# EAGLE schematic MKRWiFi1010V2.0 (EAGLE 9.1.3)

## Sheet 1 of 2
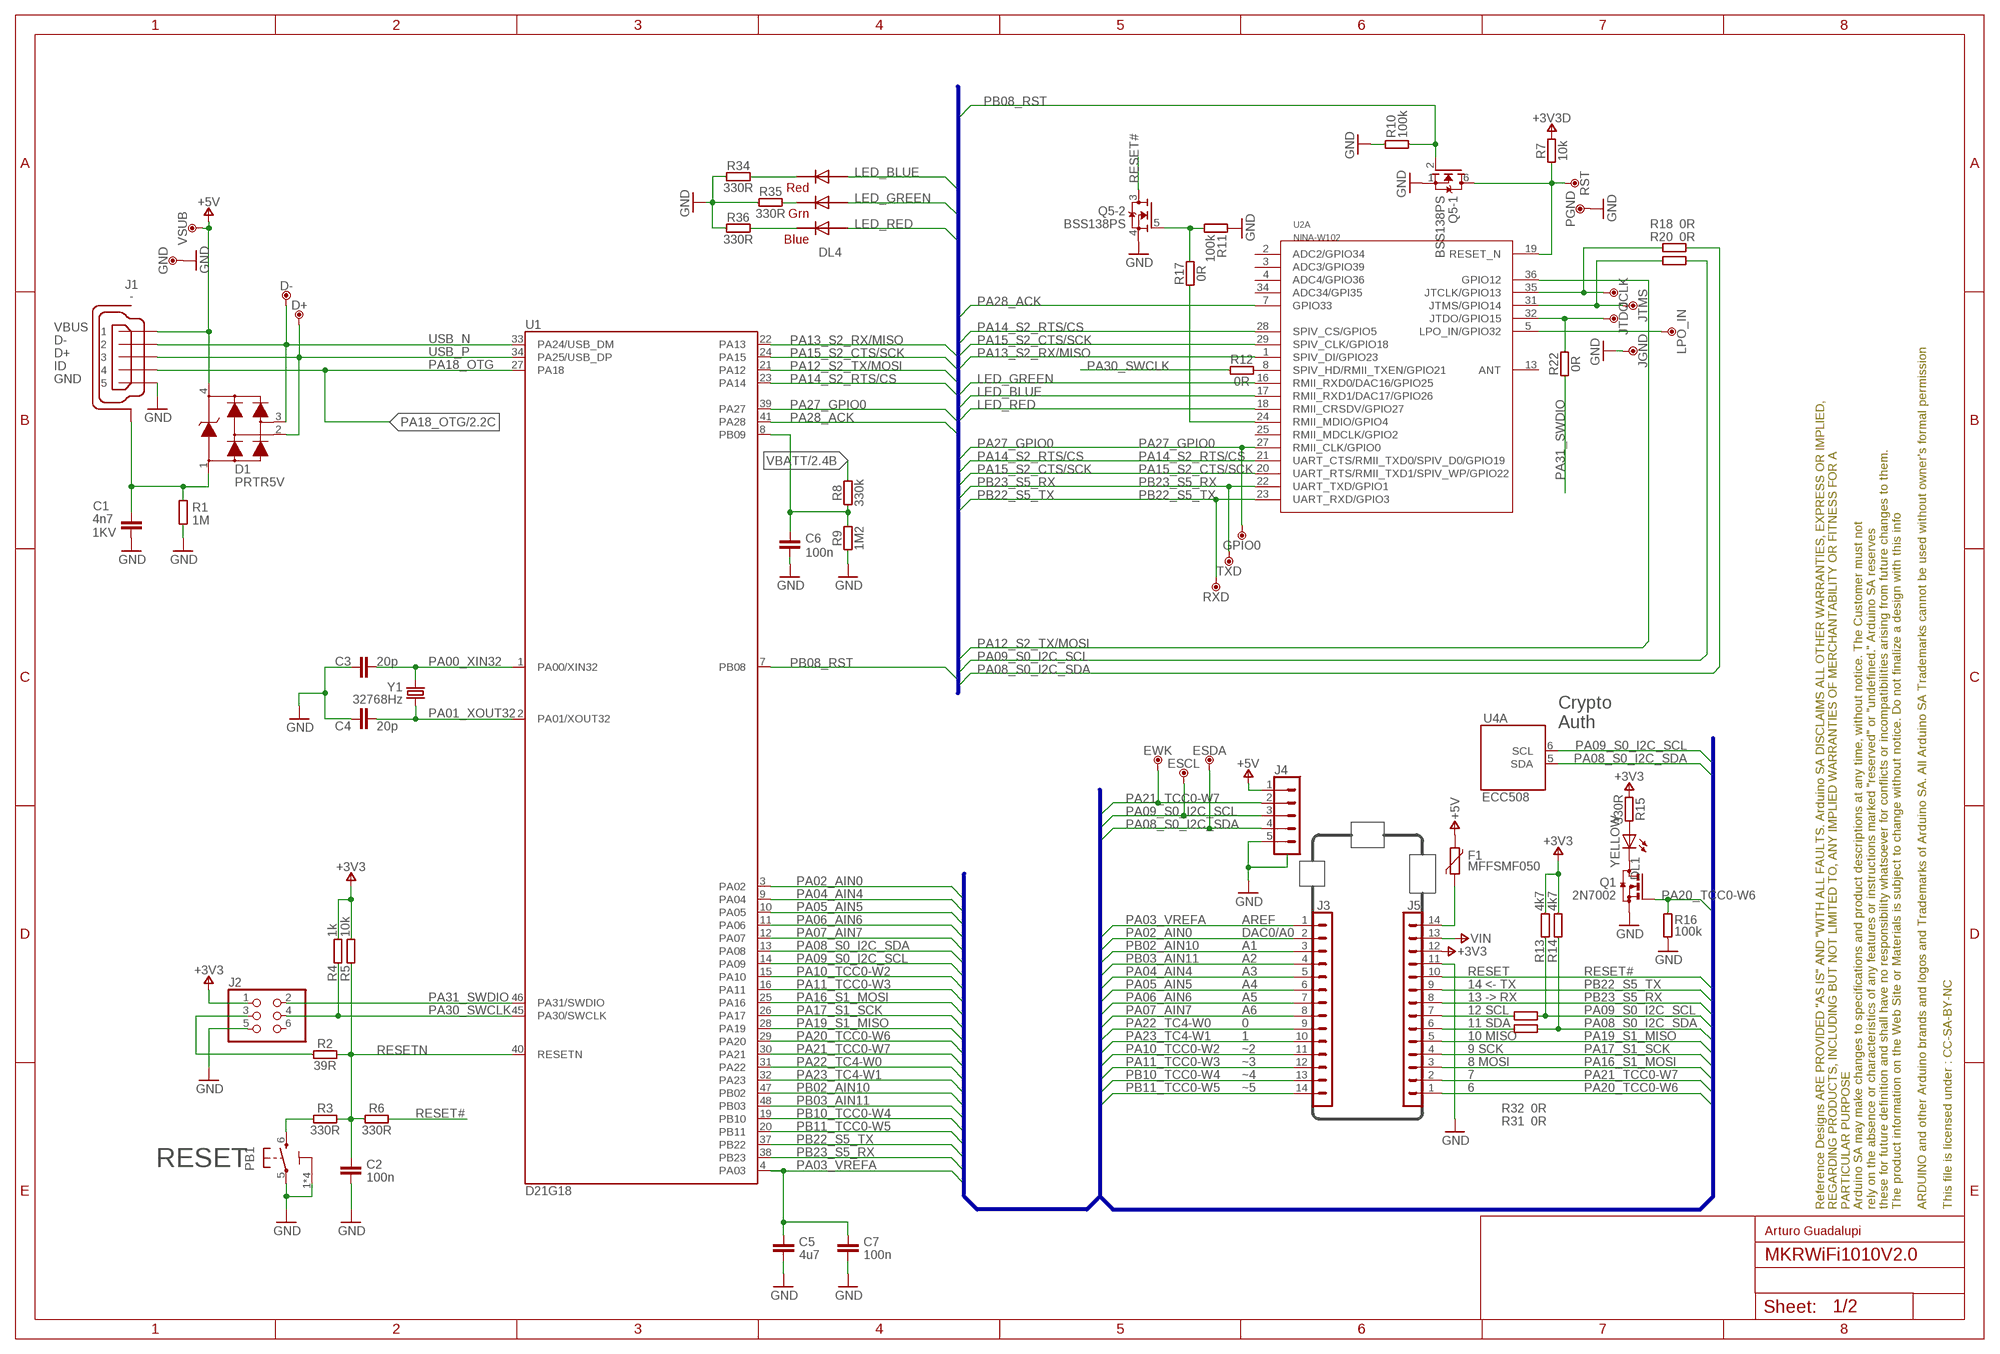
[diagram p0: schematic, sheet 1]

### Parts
C1  4n7  C4.7NF-0805  [0805-R2013X50N]
C2  100n  C-100NF-0402  [0402-1005X55N]
C3  20p  C-20PF-0402  [0402-1005X55N]
C4  20p  C-20PF-0402  [0402-1005X55N]
C5  4u7  C-4.7UF-0402  [0402-1005X55N]
C6  100n  C-100NF-0402  [0402-1005X55N]
C7  100n  C-100NF-0402  [0402-1005X55N]
D1  PRTR5V  PRTR5V0U2X,215  [SOT190P230X110-4N]
D+  DNP  TPTP-1.00MM  [TP-1.00MM]
D-  DNP  TPTP-1.00MM  [TP-1.00MM]
DL1  YELLOW  LED-YELLOW-0603  [LEDC1608X80N-AK]
DL4  RGB  RGBLED5050  [RGBLED]
ESCL  DNP  TPTP-1.00MM  [TP-1.00MM]
ESDA  DNP  TPTP-1.00MM  [TP-1.00MM]
EWK  DNP  TPTP-1.00MM  [TP-1.00MM]
F1  MFFSMF050  PTC  [0603-1608X90N]
FRAME1  DNP  A3-FRAME-STANDARD  [FRAME]
GND  DNP  TPTP-1.00MM  [TP-1.00MM]
GPIO0  DNP  TPTP-0.8MM  [TP-0.8MM]
J1  -  USB-MICRO  [ZX62-AB-5PA]
J2  DNP  PINHD-2X03-DNPSMD-NH  [2X3_SMT]
J3  -  PINHD-1X14-SM-MALE/FEMALETH-SMD  [1X14_SMD_TH]
J4  -  SM05B-SRSS-TB  [SM05B-SRSS-TB]
J5  -  PINHD-1X14-SM-MALE/FEMALETH-SMD  [1X14_SMD_TH]
JCLK  DNP  TPTP-0.8MM  [TP-0.8MM]
JGND  DNP  TPTP-0.8MM  [TP-0.8MM]
JTDO  DNP  TPTP-0.8MM  [TP-0.8MM]
JTMS  DNP  TPTP-0.8MM  [TP-0.8MM]
LPO_IN  DNP  TPTP-1.27MM  [TP-1.27MM]
PB1  PTS820  TACTILE1PTS820-NH  [C&K_PTS820_NO_HOLES]
PGND  DNP  TPTP-0.8MM  [TP-0.8MM]
Q1  2N7002  2N7002T-SOT523  [SOTFL50P160X78-3]
Q5  BSS138PS  [SOT363]
R1  1M  R-1M-0402  [0402-1005X55N]
R2  39R  R-39R-0402  [0402-1005X55N]
R3  330R  R-330R-0402  [0402-1005X55N]
R4  1k  R-1K-0402  [0402-1005X55N]
R5  10k  R-10K-0402  [0402-1005X55N]
R6  330R  R-330R-0402  [0402-1005X55N]
R7  10k  R-10K-0402  [0402-1005X55N]
R8  330k  R-330K-0402  [0402-1005X55N]
R9  1M2  R-1M2-0402  [0402-1005X55N]
R10  100k  R-100K-0402  [0402-1005X55N]
R11  100k  R-100K-0402  [0402-1005X55N]
R12  0R  R-0R-0402  [0402-1005X55N]
R13  4k7  R-4K7-0402  [0402-1005X55N]
R14  4k7  R-4K7-0402  [0402-1005X55N]
R15  330R  R-330R-0402  [0402-1005X55N]
R16  100k  R-100K-0402  [0402-1005X55N]
R17  0R  R-0R-0402  [0402-1005X55N]
R18  0R  R-0R-0402  [0402-1005X55N]
R20  0R  R-0R-0402  [0402-1005X55N]
R22  0R  R-0R-0402  [0402-1005X55N]
R31  0R  R-0R-0402  [0402-1005X55N]
R32  0R  R-0R-0402  [0402-1005X55N]
R34  330R  R-330R-0402  [0402-1005X55N]
R35  330R  R-330R-0402  [0402-1005X55N]
R36  330R  R-330R-0402  [0402-1005X55N]
RST  DNP  TPTP-0.8MM  [TP-0.8MM]
RXD  DNP  TPTP-0.8MM  [TP-0.8MM]
TXD  DNP  TPTP-0.8MM  [TP-0.8MM]
U1  D21G18  ATSAMD21G18A-48QFN  [QFN50P700X700X90-49XN-EPSQ515]
U2  NINA-W102  NINA-W1X-102  [NINA-W1X]
U4  ECC508  ATECC508A-MAHDA-T8-UDFN  [SON50P300X200X60-9N-EP160X140]
VSUB  DNP  TPTP-1.00MM  [TP-1.00MM]
Y1  32768Hz  32.768KHZ  [ABS07]

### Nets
+3V3: J2.1 J5.12 R4.2 R5.2 R13.2 R14.2 R15.1 ; also sheet 2
+3V3D: R7.2 ; also sheet 2
+5V: D1.4 F1.2 J1.1 J4.1 VSUB.X ; also sheet 2
GND: C1.2 C2.2 C3.1 C4.1 C5.2 C6.2 C7.2 GND.X J1.5 J2.5 J4.5 J4.SH1(SH) J4.SH2(SH) J5.11 JGND.X PB1.1 PB1.2 PB1.3 PB1.4 PB1.5 PGND.X Q1.S Q5.1(-1:S) Q5.4(-2:S) R1.1 R9.1 R10.2 R11.2 R16.1 R34.1 R35.1 R36.1 ; also sheet 2
LED_BLUE: DL4.2(RED_A) U2.17(A:RMII_RXD1/DAC17/GPIO26)
LED_GREEN: DL4.1(GREEN_A) U2.16(A:RMII_RXD0/DAC16/GPIO25)
LED_RED: DL4.3(BLUE_A) U2.18(A:RMII_CRSDV/GPIO27)
N17658775: PB1.6 R3.1
N$1: C1.1 D1.1 J1.6(SH) J1.7(SH) J1.8(SH) J1.9(SH) J1.10(SH) J1.11(SH) R1.2
N$2: F1.1 J5.14
N$4: J2.3 R2.1
N$5: J5.7 R32.1
N$6: C6.1 R8.1 R9.2 U1.8(PB09)
N$7: DL1.A R15.2
N$8: J5.6 R31.1
N$9: Q5.6(-1:D) R7.1 RST.X U2.19(A:RESET_N)
N$10: DL1.C Q1.D
N$11: JCLK.X R18.1 U2.35(A:JTCLK/GPIO13)
N$12: JTMS.X R20.1 U2.31(A:JTMS/GPIO14)
N$13: R17.1 U2.24(A:RMII_MDIO/GPIO4)
N$14: DL4.5(RED_C) R34.2
N$16: DL4.6(GREEN_C) R35.2
N$20: DL4.4(BLUE_C) R36.2
N$25: LPO_IN.X U2.5(A:LPO_IN/GPIO32)
N$26: JTDO.X R22.2 U2.32(A:JTDO/GPIO15)
N$27: R12.2 U2.8(A:SPIV_HD/RMII_TXEN/GPIO21)
N$28: Q5.5(-2:G) R11.1 R17.2
PA00_XIN32: C3.2 U1.1(PA00/XIN32) Y1.2
PA01_XOUT32: C4.2 U1.2(PA01/XOUT32) Y1.1
PA02_AIN0: J3.2 U1.3(PA02)
PA03_VREFA: C5.1 C7.1 J3.1 U1.4(PA03)
PA04_AIN4: J3.5 U1.9(PA04)
PA05_AIN5: J3.6 U1.10(PA05)
PA06_AIN6: J3.7 U1.11(PA06)
PA07_AIN7: J3.8 U1.12(PA07)
PA08_S0_I2C_SDA: ESDA.X J4.4 R14.1 R18.2 R31.2 U1.13(PA08) U4.5(A:SDA) ; also sheet 2
PA09_S0_I2C_SCL: ESCL.X J4.3 R13.1 R20.2 R32.2 U1.14(PA09) U4.6(A:SCL) ; also sheet 2
PA10_TCC0-W2: J3.11 U1.15(PA10)
PA11_TCC0-W3: J3.12 U1.16(PA11)
PA12_S2_TX/MOSI: U1.21(PA12) U2.36(A:GPIO12)
PA13_S2_RX/MISO: U1.22(PA13) U2.1(A:SPIV_DI/GPIO23)
PA14_S2_RTS/CS: U1.23(PA14) U2.21(A:UART_CTS/RMII_TXD0/SPIV_D0/GPIO19) U2.28(A:SPIV_CS/GPIO5)
PA15_S2_CTS/SCK: U1.24(PA15) U2.20(A:UART_RTS/RMII_TXD1/SPIV_WP/GPIO22) U2.29(A:SPIV_CLK/GPIO18)
PA16_S1_MOSI: J5.3 U1.25(PA16)
PA17_S1_SCK: J5.4 U1.26(PA17)
PA18_OTG: J1.4 U1.27(PA18) ; also sheet 2
PA19_S1_MISO: J5.5 U1.28(PA19)
PA20_TCC0-W6: J5.1 Q1.G R16.2 U1.29(PA20)
PA21_TCC0-W7: EWK.X J4.2 J5.2 U1.30(PA21)
PA22_TC4-W0: J3.9 U1.31(PA22)
PA23_TC4-W1: J3.10 U1.32(PA23)
PA27_GPIO0: GPIO0.X U1.39(PA27) U2.27(A:RMII_CLK/GPIO0)
PA28_ACK: U1.41(PA28) U2.7(A:GPIO33)
PA30_SWCLK: J2.4 R4.1 R12.1 U1.45(PA30/SWCLK)
PA31_SWDIO: J2.2 R22.1 U1.46(PA31/SWDIO)
PB02_AIN10: J3.3 U1.47(PB02)
PB03_AIN11: J3.4 U1.48(PB03)
PB08_RST: Q5.2(-1:G) R10.1 U1.7(PB08)
PB10_TCC0-W4: J3.13 U1.19(PB10)
PB11_TCC0-W5: J3.14 U1.20(PB11)
PB22_S5_TX: J5.9 RXD.X U1.37(PB22) U2.23(A:UART_RXD/GPIO3)
PB23_S5_RX: J5.8 TXD.X U1.38(PB23) U2.22(A:UART_TXD/GPIO1)
RESET#: J5.10 Q5.3(-2:D) R6.2
RESETN: C2.1 R2.2 R3.2 R5.1 R6.1 U1.40(RESETN)
USB_N [usb]: D1.3 D-.X J1.2 U1.33(PA24/USB_DM)
USB_P [usb]: D1.2 D+.X J1.3 U1.34(PA25/USB_DP)
VBATT: R8.2 ; also sheet 2
VIN: J5.13 ; also sheet 2
Unconnected: J2.6 U2.2(A:ADC2/GPIO34) U2.3(A:ADC3/GPIO39) U2.4(A:ADC4/GPIO36) U2.13(A:ANT) U2.25(A:RMII_MDCLK/GPIO2) U2.34(A:ADC34/GPI35)

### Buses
PA03_VREFA,PA02_AIN0,PB02_AIN10,PB03_AIN11,PA04_AIN4,PA05_AIN5,PA06_AIN6,PA07_AIN7,PA22_TC4-W0,PA23_TC4-W1,PA10_TCC0-W2,PA11_TCC0-W3,PB10_TCC0-W4,PB11_TCC0-W5,PA20_TCC0-W6,PA21_TCC0-W7,PA16_S1_MOSI,PA17_S1_SCK,PA19_S1_MISO,PA08_S0_I2C_SDA,PA09_S0_I2C_SCL,PB23_S5_RX,PB22_S5_TX,RESET#
B$2

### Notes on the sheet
- Crypto
  Auth
- AREF
- DAC0/A0
- A1
- A2
- A3 | RESET
- A4 | 14 <- TX
- A5 | 13 -> RX
- A6 | 12 SCL
- 0 | 11 SDA
- 1 | 10 MISO
- ~2 | 9 SCK
- ~3 | 8 MOSI
- ~4 | 7
- ~5 | 6
- RESET
- Arturo Guadalupi

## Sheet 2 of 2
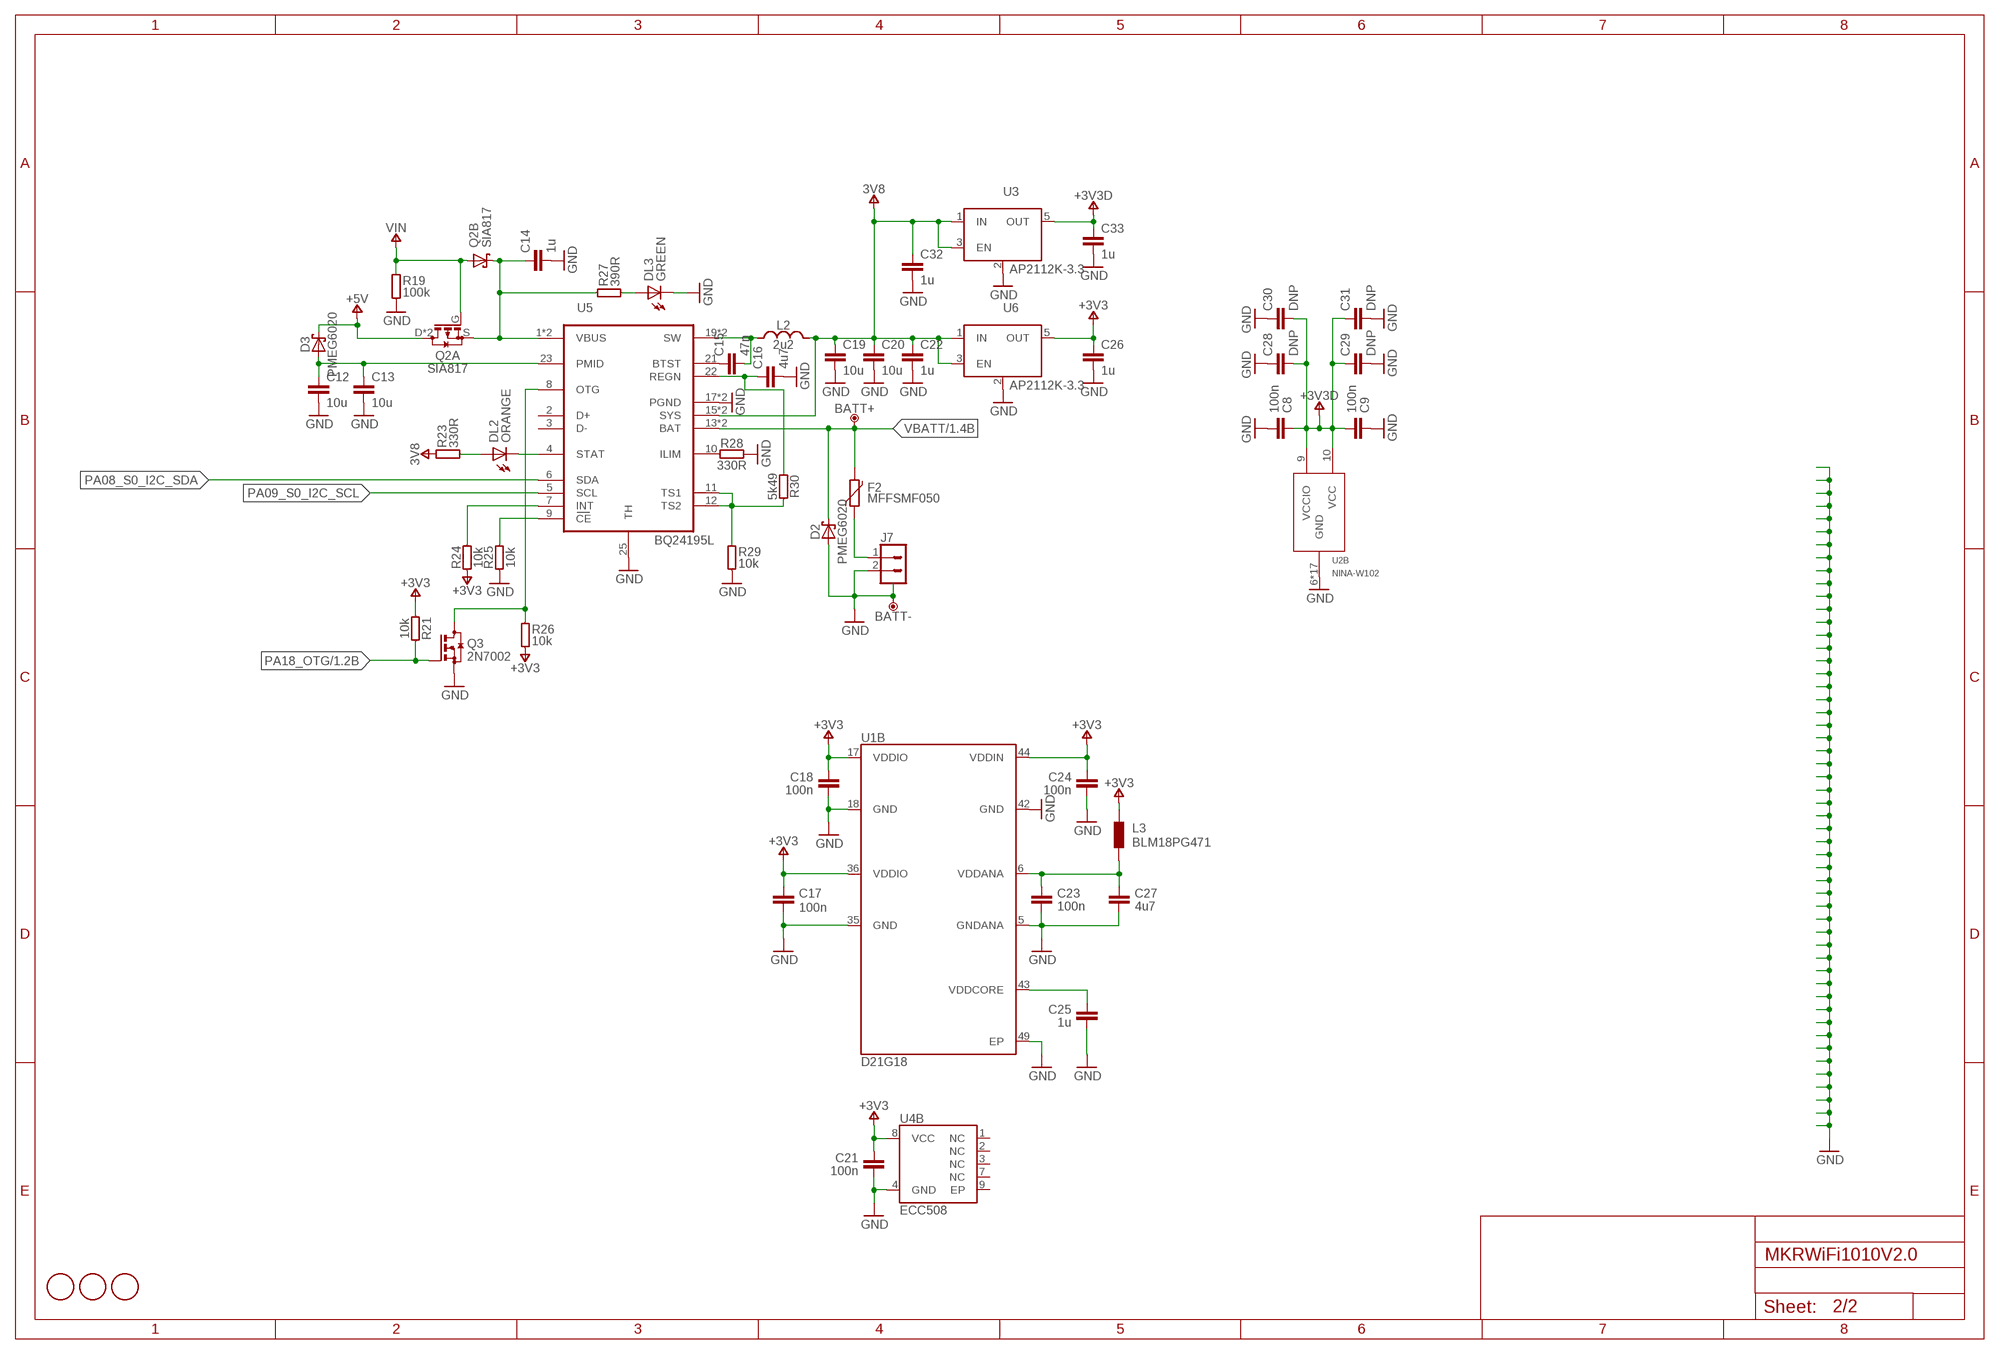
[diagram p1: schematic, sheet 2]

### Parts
BATT+  DNP  TPTP-1.00MM  [TP-1.00MM]
BATT-  DNP  TPTP-1.00MM  [TP-1.00MM]
C8  100n  C-100NF-0402  [0402-1005X55N]
C9  100n  C-100NF-0402  [0402-1005X55N]
C12  10u  C-10UF-0603  [0603-1608X90N]
C13  10u  C-10UF-0603  [0603-1608X90N]
C14  1u  C-1UF-0402  [0402-1005X55N]
C15  47n  C-47N-0402  [0402-1005X55N]
C16  4u7  C-4.7UF-0402  [0402-1005X55N]
C17  100n  C-100NF-0402  [0402-1005X55N]
C18  100n  C-100NF-0402  [0402-1005X55N]
C19  10u  C-10UF-0603  [0603-1608X90N]
C20  10u  C-10UF-0603  [0603-1608X90N]
C21  100n  C-100NF-0402  [0402-1005X55N]
C22  1u  C-1UF-0402  [0402-1005X55N]
C23  100n  C-100NF-0402  [0402-1005X55N]
C24  100n  C-100NF-0402  [0402-1005X55N]
C25  1u  C-1UF-0402  [0402-1005X55N]
C26  1u  C-1UF-0402  [0402-1005X55N]
C27  4u7  C-4.7UF-0603  [0603-1608X90N]
C28  DNP  CDNP-0402  [0402-1005X55N]
C29  DNP  CDNP-0402  [0402-1005X55N]
C30  DNP  C-DNP-0603  [0603-1608X90N]
C31  DNP  C-DNP-0603  [0603-1608X90N]
C32  1u  C-1UF-0402  [0402-1005X55N]
C33  1u  C-1UF-0402  [0402-1005X55N]
D2  PMEG6020  PMEG6020AELRX  [SODFL3517X110N]
D3  PMEG6020  PMEG6020AELRX  [SODFL3517X110N]
DL2  ORANGE  LED-ORANGE-0603  [LEDC1608X80N-AK]
DL3  GREEN  LED-GREEN-0603  [LEDC1608X80N-AK]
F2  MFFSMF050  PTC  [0603-1608X90N]
FD1  DNP  FIDUCIAL-1.5MM  [FD-1-1.5]
FD2  DNP  FIDUCIAL-1.5MM  [FD-1-1.5]
FD3  DNP  FIDUCIAL-1.5MM  [FD-1-1.5]
FRAME2  A3-FRAMEONLY  [FRAME-NO-BAN-FRAMEONLY]
J7  -  BATTERY  [JST-S2B-PH-SM4-TB]
L2  2u2  LSRP  [SRP4020]
L3  BLM18PG471  FERRITE-470R0603  [0603-1608X90N]
Q2  SIA817  SIA817EDJ  [SON65P205X205X75-8N-MWSD]
Q3  2N7002  2N7002T-SOT523  [SOTFL50P160X78-3]
R19  100k  R-100K-0402  [0402-1005X55N]
R21  10k  R-10K-0402  [0402-1005X55N]
R23  330R  R-330R-0402  [0402-1005X55N]
R24  10k  R-10K-0402  [0402-1005X55N]
R25  10k  R-10K-0402  [0402-1005X55N]
R26  10k  R-10K-0402  [0402-1005X55N]
R27  390R  R-390R-0402  [0402-1005X55N]
R28  330R  R-330R-0402  [0402-1005X55N]
R29  10k  R-10K-0402  [0402-1005X55N]
R30  5k49  R-5K49-0402  [0402-1005X55N]
U3  AP2112K-3.3  [SOT25]
U5  BQ24195L  BQ24195QFN-24  [QFN24]
U6  AP2112K-3.3  [SOT25]

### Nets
+3V3: C17.1 C18.1 C21.1 C24.1 C26.1 L3.1 R21.1 R24.1 R26.1 U1.17(VDDIO) U1.36(VDDIO) U1.44(VDDIN) U4.8(B:VCC) U6.5(OUT) ; also sheet 1
+3V3D: C8.1 C9.2 C28.2 C29.1 C30.2 C31.1 C33.1 U2.9(B:VCCIO) U2.10(B:VCC) U3.5(OUT) ; also sheet 1
+3V8: C19.1 C20.1 C22.1 C32.1 L2.2 R23.2 U3.1(IN) U3.3(EN) U5.15(SYS) U5.16(SYS) U6.1(IN) U6.3(EN) ; supply symbol labelled 3V8
+5V: D3.C Q2.D2(A:D) Q2.D(A:D) ; also sheet 1
GND: BATT-.X C8.2 C9.1 C12.2 C13.2 C14.2 C16.2 C17.2 C18.2 C19.2 C20.2 C21.2 C22.2 C23.2 C24.2 C25.2 C26.2 C27.2 C28.1 C29.2 C30.1 C31.2 C32.2 C33.2 D2.A DL3.C J7.2 J7.3(SH) J7.4(SH) Q3.S R19.1 R25.1 R28.2 R29.1 U1.5(GNDANA) U1.18(GND) U1.35(GND) U1.42(GND) U1.49(EP) U2.6(B:GND) U2.12(B:GND) U2.14(B:GND) U2.26(B:GND) U2.30(B:GND) U2.GND@1(B:GND) U2.GND@2(B:GND) U2.GND@3(B:GND) U2.GND@4(B:GND) U2.GND@5(B:GND) U2.GND@6(B:GND) U2.GND@7(B:GND) U2.GND@8(B:GND) U2.GND@9(B:GND) U2.GND@10(B:GND) U2.GND@11(B:GND) U2.GND@12(B:GND) U3.2(GND/ADJ) U4.4(B:GND) U5.17(PGND) U5.18(PGND) U5.25(TH) U6.2(GND/ADJ) ; also sheet 1
N17798864: DL2.A R23.1
N17834267: DL3.A R27.1
N17852357: C23.1 C27.1 L3.2 U1.6(VDDANA)
N17852431: C25.1 U1.43(VDDCORE)
N$3: F2.1 J7.1
N$15: C15.2 L2.1 U5.19(SW) U5.20(SW)
N$17: C14.1 Q2.K2(B:C) Q2.K(B:C) Q2.S(A:S) R27.2 U5.1(VBUS) U5.24(VBUS)
N$18: C15.1 U5.21(BTST)
N$19: R28.1 U5.10(ILIM)
N$21: C16.1 R30.1 U5.22(REGN)
N$22: Q3.D R26.2 U5.8(OTG)
N$23: R29.2 R30.2 U5.11(TS1) U5.12(TS2)
N$24: R25.2 U5.9(CE)
PA08_S0_I2C_SDA: U5.6(SDA) ; also sheet 1
PA09_S0_I2C_SCL: U5.5(SCL) ; also sheet 1
PA18_OTG: Q3.G R21.2 ; also sheet 1
PMICINT: R24.2 U5.7(INT)
STAT: DL2.C U5.4(STAT)
VBATT: BATT+.X D2.C F2.2 U5.13(BAT) U5.14(BAT) ; also sheet 1
VIN: Q2.A(B:A) Q2.G(A:G) R19.2 ; also sheet 1
VUSB1: C12.1 C13.1 D3.A U5.23(PMID)
Unconnected: U4.1(B:NC) U4.2(B:NC) U4.3(B:NC) U4.7(B:NC) U4.9(B:EP) U5.2(D+) U5.3(D-)

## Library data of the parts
BATT+ BATT- D+ D- ESCL ESDA EWK GND GPIO0 JCLK JGND JTDO JTMS LPO_IN PGND RST RXD TXD VSUB = Arduino-utility:TP: Testpoint; CODE-ARDUINO: DNP; DATASHEET: DNP; DISTRIBUTOR-LINK: DNP; DISTRIBUTOR-PN: DNP; MANUFACTURER: DNP; MANUFACTURER-PN: DNP
C1 = Arduino-rcl:C: SMD Capacitor; CODE-ARDUINO: 0689; DATASHEET: http://www.kemet.com/Lists/ProductCatalog/Attachments/40/KEM_C1010_X7R_HV_SMD.pdf; DISTRIBUTOR-LINK: www.kemet.com/docfinder?Partnumber=C0805C472KDRACTU; DISTRIBUTOR-PN: 399-6738-1-ND; MANUFACTURER: Kemet; MANUFACTURER-PN: C0805C472KDRACTU; VOLTAGE: 1KV
C2 C6-C9 C17 C18 C21 C23 C24 = Arduino-rcl:C: SMD Capacitor; CODE-ARDUINO: 0132; DATASHEET: http://www.tdk.com/pdf/TDKMLCCCapRange.pdf; DISTRIBUTOR-LINK: http://www.digikey.com/product-detail/en/tdk-corporation/C1005X5R1H104K050BB/445-5942-1-ND/2443982; DISTRIBUTOR-PN: 445-5942-1-ND; MANUFACTURER: TDK; MANUFACTURER-PN: C1005X5R1H104K050BB
C3 C4 = Arduino-rcl:C: SMD Capacitor; CODE-ARDUINO: 2188; DATASHEET: http://www.kemet.com/docfinder?Partnumber=CBR04C200J5GAC; DISTRIBUTOR-LINK: http://www.digikey.com/product-detail/en/kemet/CBR04C200J5GAC/399-6173-1-ND/2732143; DISTRIBUTOR-PN: 399-6173-1-ND; MANUFACTURER: Kemet; MANUFACTURER-PN: CBR04C200J5GAC
C5 C16 = Arduino-rcl:C: SMD Capacitor; CODE-ARDUINO: 0833; DATASHEET: http://search.murata.co.jp/Ceramy/image/img/A01X/partnumbering_e_01.pdf; DISTRIBUTOR-LINK: http://www.digikey.com/product-detail/en/murata-electronics-north-america/GRM155R60J475ME47D/490-5915-1-ND/3719860; DISTRIBUTOR-PN: 490-5915-1-ND; MANUFACTURER: Murata; MANUFACTURER-PN: GRM155R60J475ME47D
C12 C13 C19 C20 = Arduino-rcl:C: SMD Capacitor; CODE-ARDUINO: 2213; DATASHEET: http://www.murata.com/~/media/webrenewal/support/library/catalog/products/capacitor/mlcc/c02e.pdf; DISTRIBUTOR-LINK: http://www.digikey.com/product-search/en?keywords=490-10728-1-ND; DISTRIBUTOR-PN: 490-10728-1-ND; MANUFACTURER: Murata; MANUFACTURER-PN: GRM188R61C106KAALD
C14 C22 C25 C26 C32 C33 = Arduino-rcl:C: SMD Capacitor; CODE-ARDUINO: -; DATASHEET: http://search.murata.co.jp/Ceramy/image/img/A01X/partnumbering_e_01.pdf; DISTRIBUTOR-LINK: http://www.digikey.com/product-detail/en/murata-electronics-north-america/GRM155R61E105KA12D/490-10017-1-ND/5026367; DISTRIBUTOR-PN: 490-10017-1-ND; MANUFACTURER: Murata; MANUFACTURER-PN: GRM155R61E105KA12D
C15 = Arduino-rcl:C: SMD Capacitor; CODE-ARDUINO: 2216; DATASHEET: http://www.murata.com/~/media/webrenewal/support/library/catalog/products/capacitor/mlcc/c02e.pdf; DISTRIBUTOR-LINK: https://www.digikey.com/product-detail/en/murata-electronics-north-america/GRM155R71E473KA88D/490-3254-1-ND/702795; DISTRIBUTOR-PN: 490-3254-1-ND; MANUFACTURER: Murata; MANUFACTURER-PN: GRM155R71E473KA88D
C27 = Arduino-rcl:C: SMD Capacitor; CODE-ARDUINO: 0458; DATASHEET: http://www.murata.com/~/media/webrenewal/support/library/catalog/products/capacitor/mlcc/c02e.pdf; DISTRIBUTOR-LINK: http://www.digikey.com/product-search/en?keywords=490-7203-1-ND; DISTRIBUTOR-PN: 490-7203-1-ND; MANUFACTURER: Murata; MANUFACTURER-PN: GRM188R61E475KE11D
C28-C31 = Arduino-rcl:C: SMD Capacitor; CODE-ARDUINO: DNP; DATASHEET: DNP; DISTRIBUTOR-LINK: DNP; DISTRIBUTOR-PN: DNP; MANUFACTURER: DNP; MANUFACTURER-PN: DNP
D1 = Arduino-diodes:PRTR5V0U2X,215: USB ESD protection; CODE-ARDUINO: 2209; DATASHEET: http://www.nxp.com/documents/data_sheet/PRTR5V0U2X.pdf; DISTRIBUTOR-LINK: http://www.digikey.com/product-detail/en/nxp-semiconductors/PRTR5V0U2X,215/568-4140-1-ND/1589981; DISTRIBUTOR-PN: 568-4140-1-ND; MANUFACTURER: NXP; MANUFACTURER-PN: PRTR5V0U2X,215
D2 D3 = Arduino-diodes:PMEG6020AELRX: 60 V, 2 A low leakage current Schottky barrier rectifier; CODE-ARDUINO: 2208; DATASHEET: http://www.nxp.com/documents/data_sheet/PMEG6020AELR.pdf; DISTRIBUTOR-LINK: http://www.digikey.com/products/en?keywords=%20568-12710-1-ND; DISTRIBUTOR-PN: 568-12710-1-ND; MANUFACTURER: NXP; MANUFACTURER-PN: PMEG6020AELRX
DL1 = Arduino-diodes:LED: LED; CODE-ARDUINO: 2243; DATASHEET: http://media.digikey.com/pdf/Data%20Sheets/Avago%20PDFs/HSMz-Czzz.pdf; DISTRIBUTOR-LINK: http://www.digikey.com/product-detail/en/broadcom-limited/HSMY-C190/516-1424-1-ND/637748; DISTRIBUTOR-PN: 516-1424-1-ND; MANUFACTURER: Avago; MANUFACTURER-PN: HSMY-C190
DL2 = Arduino-diodes:LED: LED; CODE-ARDUINO: 2207; DATASHEET: http://media.digikey.com/pdf/Data%20Sheets/Avago%20PDFs/HSMz-Czzz.pdf; DISTRIBUTOR-LINK: http://www.digikey.com/product-detail/en/broadcom-limited/HSMD-C190/516-2489-1-ND/2744915; DISTRIBUTOR-PN: 516-2489-1-ND; MANUFACTURER: Avago; MANUFACTURER-PN: HSMD-C190
DL3 = Arduino-diodes:LED: LED; CODE-ARDUINO: 2204; DATASHEET: http://media.digikey.com/pdf/Data%20Sheets/Avago%20PDFs/HSMz-Czzz.pdf; DISTRIBUTOR-LINK: http://www.digikey.com/product-detail/en/broadcom-limited/HSMG-C190/516-1425-1-ND/637749; DISTRIBUTOR-PN: 516-1425-1-ND; MANUFACTURER: Avago; MANUFACTURER-PN: HSMG-C190
DL4 = Arduino-diodes:RGBLED: 5050 RGB LED; CODE-ARDUINO: 2211; DATASHEET: http://www.osram-os.com/Graphics/XPic9/00134830_0.pdf; DISTRIBUTOR-LINK: https://www.digikey.com/product-detail/en/osram-opto-semiconductors-inc/LTRBGFSF-ABCB-QKYO-Z/475-2899-1-ND/2415091; DISTRIBUTOR-PN: 475-2899-1-ND; MANUFACTURER: OSRAM Opto Semiconductors Inc.; MANUFACTURER-PN: LTRBGFSF-ABCB-QKYO-Z
F1 F2 = Arduino-rcl:PTC: SMD PTC; CODE-ARDUINO: 2217; DATASHEET: http://www.bourns.com/docs/Product-Datasheets/mffsmf.pdf; DISTRIBUTOR-LINK: http://www.digikey.com/product-detail/en/bourns-inc/MF-FSMF050X-2/MF-FSMF050X-2CT-ND/2039389; DISTRIBUTOR-PN: MF-FSMF050X-2CT-ND; MANUFACTURER: Bourns Inc; MANUFACTURER-PN: MF-FSMF050X-2
FD1-FD3 = Arduino-utility:FIDUCIAL: Fiducial mount; CODE-ARDUINO: DNP; DATASHEET: DNP; DISTRIBUTOR-LINK: DNP; DISTRIBUTOR-PN: DNP; MANUFACTURER: DNP; MANUFACTURER-PN: DNP
FRAME1 = Arduino-utility:A3-FRAME: Schematic frame; CODE-ARDUINO: DNP; DATASHEET: DNP; DISTRIBUTOR-LINK: DNP; DISTRIBUTOR-PN: DNP; MANUFACTURER: DNP; MANUFACTURER-PN: DNP
FRAME2 = Arduino-utility:A3-FRAMEONLY: Schematic frame
J1 = Arduino-connectors:USB-MICRO: USB - micro AB USB 2.0 Receptacle Connector 5 Position Surface Mount, Right Angle, Horizontal; CODE-ARDUINO: 2219; DATASHEET: https://www.hirose.com/product/en/download_file/key_name/ZX/category/Catalog/doc_file_id/31704/?file_category_id=4&item_id=13&is_series=1; DISTRIBUTOR-LINK: http://www.digikey.com/product-detail/en/hirose-electric-co-ltd/ZX62-AB-5PA(31)/H125279CT-ND/5994741; DISTRIBUTOR-PN: H125279CT-ND; MANUFACTURER: Hirose; MANUFACTURER-PN: ZX62-AB-5PA(31)
J2 = Arduino-connectors:PINHD-2X03: PIN HEADER; CODE-ARDUINO: DNP; DATASHEET: DNP; DISTRIBUTOR-LINK: DNP; DISTRIBUTOR-PN: DNP; MANUFACTURER: DNP; MANUFACTURER-PN: DNP
J3 J5 = Arduino-connectors:PINHD-1X14-SM: PIN HEADER; CODE-ARDUINO: -; DATASHEET: -; DISTRIBUTOR-LINK: -; DISTRIBUTOR-PN: -; MANUFACTURER: ELDECO; MANUFACTURER-PN: FH254114DF08500T
J4 = Arduino-connectors:SM05B-SRSS-TB: CONN HEADER SH 5POS SIDE 1MM TIN Datasheet; CODE-ARDUINO: 2353; DATASHEET: http://www.jst-mfg.com/product/pdf/eng/eSH.pdf; DISTRIBUTOR-LINK: http://www.digikey.com/product-detail/en/jst-sales-america-inc/SM05B-SRSS-TB(LF)(SN)/455-1805-1-ND/926876; DISTRIBUTOR-PN: 455-1805-1-ND; MANUFACTURER: JST; MANUFACTURER-PN: SM05B-SRSS-TB
J7 = Arduino-connectors:BATTERY: CONN HEADER PH SIDE 2POS 2MM SMD; CODE-ARDUINO: 2355; DATASHEET: http://www.jst-mfg.com/product/pdf/eng/ePH.pdf; DISTRIBUTOR-LINK: http://www.digikey.com/product-detail/en/jst-sales-america-inc/S2B-PH-SM4-TB%28LF%29%28SN%29/455-1749-1-ND/926846; DISTRIBUTOR-PN: 455-1749-1-ND; MANUFACTURER: JST; MANUFACTURER-PN: S2B-PH-SM4-TB(LF)(SN)
L2 = Arduino-rcl:L: Inductors; CODE-ARDUINO: 2218; DATASHEET: http://www.bourns.com/docs/Product-Datasheets/SRP4020TA.pdf; DISTRIBUTOR-LINK: https://www.digikey.com/product-detail/en/bourns-inc/SRP4020TA-2R2M/SRP4020TA-2R2MCT-ND/4901068; DISTRIBUTOR-PN: SRP4020TA-2R2MCT-ND; MANUFACTURER: Bourns; MANUFACTURER-PN: SRP4020TA-2R2M
L3 = Arduino-rcl:FERRITE: SMD ferrite; CODE-ARDUINO: 2217; DATASHEET: http://search.murata.co.jp/Ceramy/image/img/PDF/ENG/L0110S0100BLM18P.pdf; DISTRIBUTOR-LINK: http://www.digikey.com/product-detail/en/murata-electronics-north-america/BLM18PG471SN1D/490-5223-1-ND/1948399; DISTRIBUTOR-PN: 490-5223-1-ND; MANUFACTURER: Murata; MANUFACTURER-PN: BLM18PG471SN1D
PB1 = Arduino-pushbuttons:TACTILE1: Tactile Switch SPST-NO Top Actuated Surface Mount; CODE-ARDUINO: 0277; DATASHEET: http://www.ckswitches.com/media/1474/pts820.pdf; DISTRIBUTOR-LINK: https://www.digikey.com/product-detail/en/c-k/PTS820-J15M-SMTR-LFS/CKN10506CT-ND/4176681; DISTRIBUTOR-PN: PTS820 J25K SMTR LFS-ND; MANUFACTURER: C&K; MANUFACTURER-PN: PTS820 J25K SMTR LFS
Q1 Q3 = Arduino-transistors:2N7002T: MOSFET N-CH 60V 115MA; CODE-ARDUINO: 1612; DATASHEET: http://www.diodes.com/_files/datasheets/ds30301.pdf; DISTRIBUTOR-LINK: http://www.digikey.com/product-detail/en/diodes-incorporated/2N7002T-7-F/2N7002T-FDICT-ND/815290; DISTRIBUTOR-PN: 2N7002T-FDICT-ND; MANUFACTURER: Diodes Incorporated; MANUFACTURER-PN: 2N7002T-7-F
Q2 = Arduino-transistors:SIA817EDJ: MOSFET P-CH 30V 4.5A SC-70-6; CODE-ARDUINO: 2220; DATASHEET: http://www.vishay.com/docs/62820/sia817edj.pdf; DISTRIBUTOR-LINK: http://www.digikey.com/product-detail/en/vishay-siliconix/SIA817EDJ-T1-GE3/SIA817EDJ-T1-GE3CT-ND/4142098; DISTRIBUTOR-PN: SIA817EDJ-T1-GE3CT-ND; MANUFACTURER: Vishay; MANUFACTURER-PN: SIA817EDJ-T1-GE3
Q5 = Arduino-transistors:BSS138PS: MOSFET 2N-CH 60V 0.32A 6TSSOP; DATASHEET: http://www.nxp.com/documents/data_sheet/BSS138PS.pdf; DISTRIBUTOR-LINK: http://www.digikey.com/product-detail/en/nxp-semiconductors/BSS138PS,115/568-8393-1-ND/2763927; DISTRIBUTOR-PN: 568-8393-1-ND; MANUFACTURER: NXP; MANUFACTURER-PN: BSS138PS,115
R1 = Arduino-rcl:R: SMD Resistor; CODE-ARDUINO: 0139; DATASHEET: www.yageo.com.tw/exep/pages/download/literatures/PYu-R_INT-thick_7.pdf; DISTRIBUTOR-LINK: http://www.digikey.com/product-detail/en/yageo/RC0402JR-07330RL/311-330JRCT-ND/729412; DISTRIBUTOR-PN: 311-330JRCT-ND; MANUFACTURER: Yageo; MANUFACTURER-PN: RC0402JR-07330RL
R2 = Arduino-rcl:R: SMD Resistor; CODE-ARDUINO: 0138; DATASHEET: www.yageo.com.tw/exep/pages/download/literatures/PYu-R_INT-thick_7.pdf; DISTRIBUTOR-LINK: http://www.digikey.com/product-detail/en/yageo/RC0402FR-0739RL/311-39.0LRCT-ND/729549; DISTRIBUTOR-PN: 311-39.0LRCT-ND; MANUFACTURER: Yageo; MANUFACTURER-PN: RC0402FR-0739RL
R3 R6 R15 R23 R28 R34-R36 = Arduino-rcl:R: SMD Resistor; CODE-ARDUINO: 2229; DATASHEET: www.yageo.com.tw/exep/pages/download/literatures/PYu-R_INT-thick_7.pdf; DISTRIBUTOR-LINK: http://www.digikey.com/product-detail/en/yageo/RC0402FR-07330RL/311-330LRCT-ND/729541; DISTRIBUTOR-PN: 311-330LRCT-ND; MANUFACTURER: Yageo; MANUFACTURER-PN: RC0402FR-07330RL
R4 = Arduino-rcl:R: SMD Resistor; CODE-ARDUINO: 0140; DATASHEET: www.yageo.com.tw/exep/pages/download/literatures/PYu-R_INT-thick_7.pdf; DISTRIBUTOR-LINK: http://www.digikey.com/product-detail/en/yageo/RC0402FR-071KL/311-1.00KLRCT-ND/729460; DISTRIBUTOR-PN: 311-1.00KLRCT-ND; MANUFACTURER: Yageo; MANUFACTURER-PN: RC0402FR-071KL
R5 R7 R21 R24-R26 R29 = Arduino-rcl:R: SMD Resistor; CODE-ARDUINO: 0136; DATASHEET: www.yageo.com.tw/exep/pages/download/literatures/PYu-R_INT-thick_7.pdf; DISTRIBUTOR-LINK: http://www.digikey.com/product-detail/en/yageo/RC0402FR-0710KL/311-10.0KLRCT-ND/729470; DISTRIBUTOR-PN: 311-10.0KLRCT-ND; MANUFACTURER: Yageo; MANUFACTURER-PN: RC0402FR-0710KL
R8 = Arduino-rcl:R: SMD Resistor; CODE-ARDUINO: 2192; DATASHEET: www.yageo.com.tw/exep/pages/download/literatures/PYu-R_INT-thick_7.pdf; DISTRIBUTOR-LINK: http://www.digikey.com/product-detail/en/yageo/RC0402JR-07330KL/311-330KJRCT-ND/729413; DISTRIBUTOR-PN: 311-330KJRCT-ND; MANUFACTURER: Yageo; MANUFACTURER-PN: RC0402JR-07330KL
R9 = Arduino-rcl:R: SMD Resistor; CODE-ARDUINO: 2352; DATASHEET: www.yageo.com.tw/exep/pages/download/literatures/PYu-R_INT-thick_7.pdf; DISTRIBUTOR-LINK: http://www.digikey.com/products/en?keywords=RC0402FR-071M2L-ND; DISTRIBUTOR-PN: RC0402FR-071M2L-ND; MANUFACTURER: Yageo; MANUFACTURER-PN: RC0402FR-071M2L
R10 R11 R16 R19 = Arduino-rcl:R: SMD Resistor; CODE-ARDUINO: 0134; DATASHEET: www.yageo.com.tw/exep/pages/download/literatures/PYu-R_INT-thick_7.pdf; DISTRIBUTOR-LINK: http://www.digikey.com/product-detail/en/yageo/RC0402FR-07100KL/311-100KLRCT-ND/729473; DISTRIBUTOR-PN: 311-100KLRCT-ND; MANUFACTURER: Yageo; MANUFACTURER-PN: RC0402FR-07100KL
R12 R17 R18 R20 R22 R31 R32 = Arduino-rcl:R: SMD Resistor; CODE-ARDUINO: 0039; DATASHEET: www.yageo.com.tw/exep/pages/download/literatures/PYu-R_INT-thick_7.pdf; DISTRIBUTOR-LINK: http://www.digikey.com/product-detail/en/yageo/RC0402FR-070RL/311-0.0LRCT-ND/2827888; DISTRIBUTOR-PN: 311-0.0LRCT-ND; MANUFACTURER: Yageo; MANUFACTURER-PN: RC0402FR-070RL
R13 R14 = Arduino-rcl:R: SMD Resistor; CODE-ARDUINO: 2196; DATASHEET: www.yageo.com.tw/exep/pages/download/literatures/PYu-R_INT-thick_7.pdf; DISTRIBUTOR-LINK: http://www.digikey.com/product-detail/en/yageo/RC0402FR-074K7L/311-4.7KLRCT-ND/2827881; DISTRIBUTOR-PN: 311-4.7KLRCT-ND; MANUFACTURER: Yageo; MANUFACTURER-PN: RC0402FR-074K7L
R27 = Arduino-rcl:R: SMD Resistor; CODE-ARDUINO: 2195; DATASHEET: www.yageo.com.tw/exep/pages/download/literatures/PYu-R_INT-thick_7.pdf; DISTRIBUTOR-LINK: https://www.digikey.com/product-detail/en/yageo/RC0402FR-07390RL/311-390LRCT-ND/2827929; DISTRIBUTOR-PN: 311-390LRCT-ND; MANUFACTURER: Yageo; MANUFACTURER-PN: RC0402FR-07390RL
R30 = Arduino-rcl:R: SMD Resistor; CODE-ARDUINO: 2197; DATASHEET: www.yageo.com.tw/exep/pages/download/literatures/PYu-R_INT-thick_7.pdf; DISTRIBUTOR-LINK: https://www.digikey.com/product-detail/en/yageo/RC0402FR-075K49L/311-5.49KLRCT-ND/729573; DISTRIBUTOR-PN: 311-5.49KLRCT-ND; MANUFACTURER: Yageo; MANUFACTURER-PN: RC0402FR-075K49L
U1 = Arduino-ucs&SoCs:ATSAMD21G18A-48: ARM® Cortex®-M0+ SAM D21G Microcontroller IC 32-Bit 48MHz 256KB (256K x 8) FLASH 48-TQFP (7x7); CODE-ARDUINO: 2202; DATASHEET: http://www.atmel.com/Images/Atmel-42181-SAM-D21_Datasheet.pdf; DISTRIBUTOR-LINK: https://www.digikey.com/product-detail/en/microchip-technology/ATSAMD21G18A-MU/ATSAMD21G18A-MU-ND/4935894; DISTRIBUTOR-PN: ATSAMD21G18A-MU-ND; MANUFACTURER: Atmel; MANUFACTURER-PN: ATSAMD21G18A-MU
U2 = Arduino-ucs&SoCs:NINA-W1X: ESP32 WiFi/BLE module; CODE-ARDUINO: 2205; DATASHEET: https://www.u-blox.com/sites/default/files/NINA-W1_DataSheet_%28UBX-17006694%29.pdf; DISTRIBUTOR-LINK: https://www.digikey.com/product-detail/en/u-blox-america-inc/NINA-W102/672-1070-1-ND/7931820; DISTRIBUTOR-PN: 672-1070-1-ND; MANUFACTURER: Ublocks; MANUFACTURER-PN: NINA-W102
U3 U6 = Arduino-ICs:AP2112K-3.3: IC REG LINEAR 3.3V 600mA SOT25; CODE-ARDUINO: 2199; DATASHEET: https://www.diodes.com/assets/Datasheets/AP2112.pdf; DISTRIBUTOR-LINK: https://www.digikey.com/product-detail/en/diodes-incorporated/AP2112K-3.3TRG1/AP2112K-3.3TRG1DITR-ND/4470746; DISTRIBUTOR-PN: AP2112K-3.3TRG1DITR-ND; MANUFACTURER: Diodes Inc; MANUFACTURER-PN: AP2112K-3.3TRG1
U4 = Arduino-ICs:ATECC508A-MAHDA-T: Secure authentication and product validation device, EEPROM, I2C, 2.0 - 5.5V; CODE-ARDUINO: 2203; DATASHEET: http://www.atmel.com/Images/Atmel-8923S-CryptoAuth-ATECC508A-Datasheet-Summary.pdf; DISTRIBUTOR-LINK: http://www.digikey.com/product-detail/en/atmel/ATECC508A-MAHDA-T/ATECC508A-MAHDA-TCT-ND/5213071; DISTRIBUTOR-PN: ATECC508A-MAHDA-TCT-ND; MANUFACTURER: Atmel; MANUFACTURER-PN: ATECC508A-MAHDA-T
U5 = Arduino-ICs:BQ24195: IC CHRG MGMT LI-ION/POL; CODE-ARDUINO: 2201; DATASHEET: http://www.ti.com/lit/ds/symlink/bq24195.pdf; DISTRIBUTOR-LINK: https://www.digikey.com/product-detail/en/texas-instruments/BQ24195LRGET/296-35047-1-ND/3725759; DISTRIBUTOR-PN: 296-35047-1-ND; MANUFACTURER: Texas Instruments; MANUFACTURER-PN: BQ24195LRGET
Y1 = Arduino-crystals:32.768KHZ: LF crystal; CODE-ARDUINO: 0213; DATASHEET: http://www.abracon.com/Resonators/ABS07.pdf; DISTRIBUTOR-LINK: http://www.digikey.com/product-detail/en/abracon-llc/ABS07-32.768KHZ-T/535-9542-1-ND/1237009; DISTRIBUTOR-PN: 535-9542-1-ND; MANUFACTURER: Abracon LLC; MANUFACTURER-PN: ABS07-32.768KHZ-T

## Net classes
0 default: width 0.19 mm, drill 0.19 mm
1 usb: width 0.19 mm, drill 0.19 mm, clearance 0.127 mm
